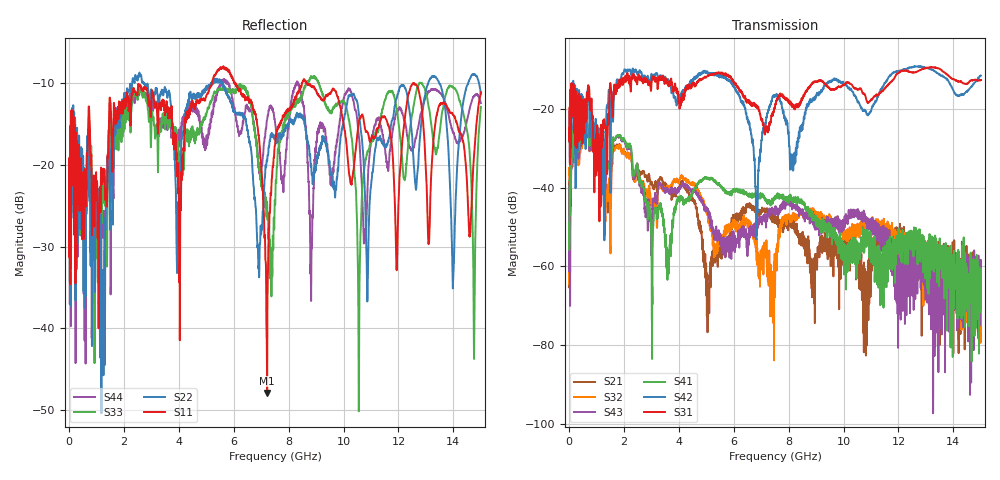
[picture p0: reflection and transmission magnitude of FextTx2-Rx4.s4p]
! FILE: N:\QM 2007\Prüfprotokolle\Highspeed\Konfektionierte Ltg\L45593-D106\D30\8216\0002\Fext\FextTx2-Rx4.s4p
# MHz S RI R 50.00
! FREQ  S11  S12  S13  S14
!  S21  S22  S23  S24
!  S31  S32  S33  S34
!  S41  S42  S43  S44
!  REAL  IMAG  REAL  IMAG  REAL  IMAG  REAL  IMAG
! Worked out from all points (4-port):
!   2999 points, 10 MHz to 15 GHz, reference 50 ohm
!   strongest paths, dB at 10 MHz, 3.755 GHz, 7.505 GHz, 11.26 GHz, 15 GHz:
!     S31: -24.8, -13.3, -19.3, -16.3, -12.6
!     S42: -25.1, -15.4, -16.9, -16.9, -11.5
!     S41: -48.9, -49.9, -42.2, -57.0, -60.8
!     S43: -41.2, -40.2, -45.0, -51.9, -69.8
!     S32: -34.9, -39.4, -67.8, -49.8, -69.0
!     S21: -46.1, -42.5, -47.8, -54.9, -65.6
!   lowest |S11| = -47.9 dB at 7.22 GHz (marker M1), VSWR 1.01, Z = 50.3 + j0.222 ohm
!   |S11| at or under -10 dB: start of sweep to 5.212 GHz; 8.672 GHz to 12.53 GHz (3.859 GHz wide, 36.4 % of centre); 12.56 GHz to end of sweep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
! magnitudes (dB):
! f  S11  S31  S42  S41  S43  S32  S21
! 10 MHz  -19.4  -24.8  -25.1  -48.9  -41.2  -34.9  -46.1
! 610 MHz  -25.1  -22.9  -30.1  -21.9  -23.4  -23.7  -22.9
! 3.61 GHz  -14.2  -13.0  -12.4  -60.7  -40.8  -40.5  -40.1
! 5.685 GHz  -8.2  -10.9  -11.9  -40.9  -55.7  -50.4  -54.6
! 6.84 GHz  -14.5  -19.6  -52.0  -41.6  -49.9  -58.5  -46.0
! 7.22 GHz  -47.9  -24.7  -21.1  -43.3  -47.5  -58.3  -45.6
! 15 GHz  -11.1  -12.6  -11.5  -60.8  -69.8  -69.0  -65.6
